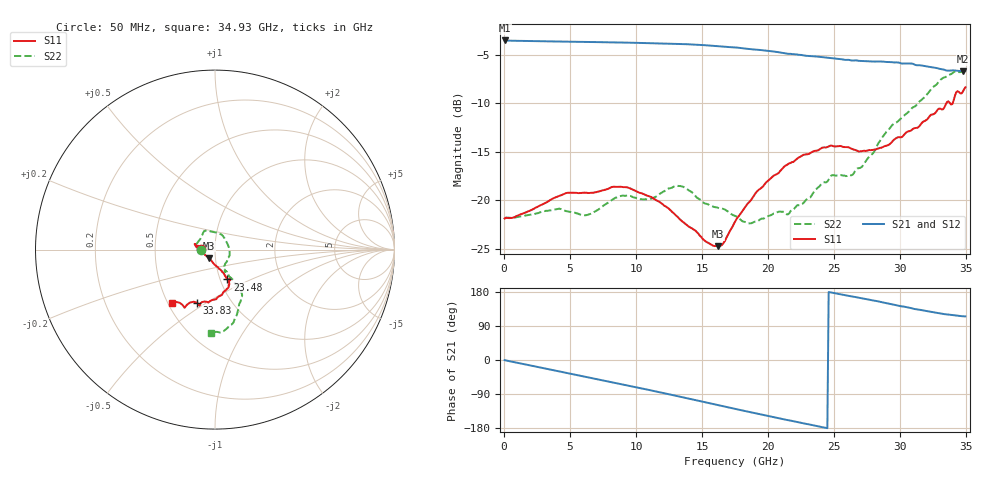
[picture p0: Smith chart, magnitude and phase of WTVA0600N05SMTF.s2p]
! 50 ohm 2-Port S-parameters measured by Modelithics Inc support@modelithics.com  Tampa, FL USA 813-866-6335 (February 2024)
! Smiths Interconnect,  6dB P/N: WTVA0600N05SMTF, Temperature: 125 C
! Board: 10 mil Rogers 4350B, Mounting Pad Dimensions: Length: 15 mils, Width: 25 mils, Gap: 40 mils.
# Hz S RI R 50
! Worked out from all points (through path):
!   352 points, 50 MHz to 34.93 GHz, reference 50 ohm
!   highest |S21| = -3.51 dB at 100 MHz (marker M1); lowest = -6.7 dB at 34.73 GHz (marker M2)
!   group delay of S21, straight-line fit = 20.1 ps
!   lowest |S11| = -24.7 dB at 16.22 GHz (marker M3), VSWR 1.12, Z = 46.4 - j4.3 ohm
!   |S11| at or under -10 dB: start of sweep to 33.48 GHz; 33.77 GHz to 33.95 GHz (179.5 MHz wide, 0.53 % of centre)
!   |S22| runs from -22.4 to -6.7 dB; largest |S21 - S12| = 0.007
!   S11 on the Smith chart (normalised r, x): 50 MHz: 0.85, +0.00; 23.48 GHz: 1.08, -0.37; 33.83 GHz: 0.70, -0.46; 34.93 GHz: 0.52, -0.37
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5e7  -0.0807 0.00137  0.6677 -0.0043  0.6669 -0.00405  -0.0801 -0.000648
1e8  -0.0811 0.00122  0.6678 -0.00907  0.6668 -0.00911  -0.0812 0.000228
2.986e9  -0.0935 0.0212  0.6156 -0.2416  0.6143 -0.242  -0.0874 0.0104
5.8715e9  -0.1051 0.0298  0.4879 -0.44  0.4871 -0.4396  -0.0833 0.0118
9.155e9  -0.1131 0.0303  0.2676 -0.5935  0.2668 -0.5927  -0.0998 0.0343
1.1742e10  -0.098 0.00996  0.0588 -0.6417  0.0571 -0.641  -0.0721 0.0795
1.34335e10  -0.0784 -0.00367  -0.0846 -0.6347  -0.0863 -0.6335  -0.0537 0.1053
1.62195e10  -0.0351 -0.0462  -0.3031 -0.545  -0.3038 -0.5437  0.0274 0.0872
1.7513e10  -0.00805 -0.0776  -0.3865 -0.4778  -0.3867 -0.4764  0.0525 0.0643
1.8508e10  0.0136 -0.0961  -0.4388 -0.4154  -0.4392 -0.414  0.0683 0.0333
2.1493e10  0.0539 -0.1437  -0.531 -0.2074  -0.5307 -0.2056  0.0703 -0.0472
2.33835e10  0.0674 -0.1655  -0.5485 -0.0766  -0.5477 -0.0762  0.0521 -0.0954
2.3483e10  0.0691 -0.166  -0.549 -0.0702  -0.5482 -0.069  0.0531 -0.0976
2.47765e10  0.0787 -0.175  -0.5412 0.0181  -0.5403 0.0196  0.058 -0.121
2.63685e10  0.0844 -0.1635  -0.5138 0.1132  -0.5126 0.1144  0.0616 -0.1204
2.91545e10  0.0778 -0.1777  -0.4414 0.2693  -0.4378 0.2733  0.1242 -0.1976
3.1841e10  0.0358 -0.2539  -0.3171 0.3768  -0.3142 0.3778  0.1328 -0.3138
3.35325e10  -0.0859 -0.3095  -0.2364 0.4026  -0.2325 0.404  0.0736 -0.431
3.3831e10  -0.0997 -0.296  -0.2274 0.4085  -0.2235 0.4096  0.0612 -0.4434
3.4229e10  -0.1667 -0.3198  -0.2151 0.4137  -0.2108 0.415  0.0274 -0.4619
3.47265e10  -0.2151 -0.2922  -0.2002 0.4182  -0.199 0.4178  -0.0133 -0.4604
3.49255e10  -0.2411 -0.2979  -0.1973 0.4214  -0.196 0.4208  -0.0244 -0.4621
